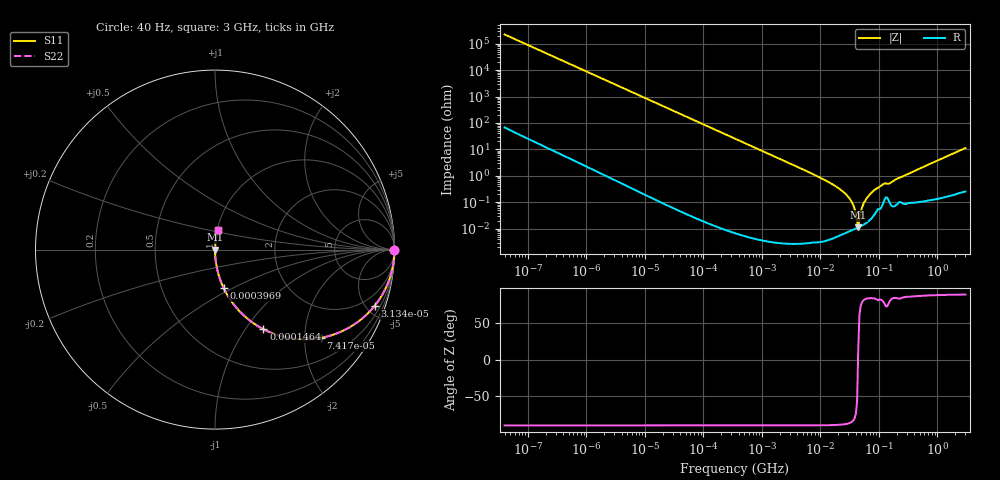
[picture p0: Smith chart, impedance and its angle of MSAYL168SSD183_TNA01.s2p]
! MSAYL168SSD183_TNA01  S-PARAMETER MODEL  ( General Type )
! Model Generated by TAIYO YUDEN Corporation (http://www.ty-top.com)
! Version 2.0
! TAIYO YUDEN Control No. 031107
! Copyright(c) 2003 TAIYO YUDEN CO.,LTD. All Rights Reserved.
! Product Description (link to TY-COMPAS)
! https://ds.yuden.co.jp/TYCOMPAS/or/detail?pn=MSAYL168SSD183KTNA01&u=M
! Products Name : Multilayer Ceramic Capacitors
! Characteristics :
!  Capacitance : 0.018 uF , Rated Voltage : 10V
!  Case Size : 1.6 x 0.8 / 0.063 x 0.031 [mm/inch] , Thickness : 0.8 / 0.031 [mm/inch]
!  (Conditions: Temperature = 25 degC , DC Bias Current/Voltage = 0A / 0V)
! External Node Assignments :
!  1  o---| |---o  2
! GND o---------o GND
! Frequency Range : 40Hz  -  3GHz  [ 401 STEP ]
# MHz S RI R 50
! Freq[MHz].  S11 Real  S11 Imag  S21 Real  S21 Imag  S12 Real  S12 Imag  S22 Real  S22 Imag
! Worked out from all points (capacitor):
!   401 points, 40 Hz to 3 GHz, reference 50 ohm
!   read as one part in series: C = 17.9 nF near 44 Hz
!   lowest |Z| = 11.5 mohm at 44.28 MHz (marker M1)
!   series resonance near 43.97 MHz, so ESL is about 730 pH
!   S11 on the Smith chart (normalised r, x): 40 Hz: open; 31.34 kHz: 1.00, -5.67; 74.17 kHz: 1.00, -2.40; 146.4 kHz: 1.00, -1.21; 396.9 kHz: 1.00, -0.45; 3 GHz: 1.01, +0.22
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4e-05  1 -0.00045  3.39e-07 0.00045  3.39e-07 0.00045  1 -0.00045
0.000834  0.9999 -0.00938  9.04e-05 0.00938  9.04e-05 0.00938  0.9999 -0.00938
0.017386  0.9631 -0.1883  0.0369 0.1883  0.0369 0.1883  0.9631 -0.1883
0.031343  0.8894 -0.3135  0.1106 0.3135  0.1106 0.3135  0.8894 -0.3135
0.074167  0.5897 -0.4918  0.4103 0.4918  0.4103 0.4918  0.5897 -0.4918
0.146395  0.2695 -0.4436  0.7305 0.4436  0.7305 0.4436  0.2695 -0.4436
0.362475  0.0568 -0.2313  0.9432 0.2313  0.9432 0.2313  0.0568 -0.2313
0.396875  0.0478 -0.2133  0.9522 0.2133  0.9522 0.2133  0.0478 -0.2133
1.28983  0.00475 -0.0686  0.9952 0.0686  0.9952 0.0686  0.00475 -0.0686
7.222098  0.000173 -0.012  0.9998 0.012  0.9998 0.012  0.000173 -0.012
16.33207  6.47e-05 -0.00468  0.9999 0.00468  0.9999 0.00468  6.47e-05 -0.00468
26.8909  7.28e-05 -0.00206  0.9999 0.00206  0.9999 0.00206  7.28e-05 -0.00206
33.73212  8.63e-05 -0.00108  0.9999 0.00108  0.9999 0.00108  8.63e-05 -0.00108
36.93337  9.33e-05 -0.000712  0.9999 0.000712  0.9999 0.000712  9.33e-05 -0.000712
40.43842  0.000101 -0.000337  0.9999 0.000337  0.9999 0.000337  0.000101 -0.000337
44.27611  0.000111 2.86e-05  0.9999 -2.86e-05  0.9999 -2.86e-05  0.000111 2.86e-05
46.32945  0.000116 0.000206  0.9999 -0.000206  0.9999 -0.000206  0.000116 0.000206
55.54024  0.000146 0.000953  0.9999 -0.000953  0.9999 -0.000953  0.000146 0.000953
69.67004  0.000215 0.00194  0.9998 -0.00194  0.9998 -0.00194  0.000215 0.00194
114.7124  0.000803 0.00456  0.9992 -0.00456  0.9992 -0.00456  0.000803 0.00456
150.5692  0.00103 0.00502  0.999 -0.00502  0.999 -0.00502  0.00103 0.00502
3000  0.0149 0.1103  0.9851 -0.1103  0.9851 -0.1103  0.0149 0.1103
